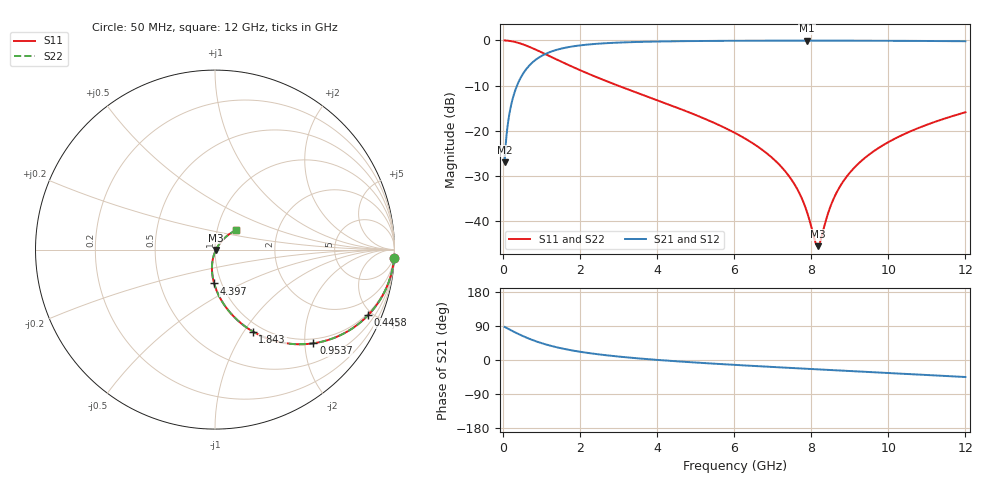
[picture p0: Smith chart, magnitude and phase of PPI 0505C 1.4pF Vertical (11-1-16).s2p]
# GHz S MA R 50
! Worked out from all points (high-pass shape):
!   1601 points, 50 MHz to 12 GHz, reference 50 ohm
!   highest |S21| = -0.05 dB at 7.892 GHz (marker M1); lowest = -27.0 dB at 50 MHz (marker M2)
!   |S21| within 3 dB of the highest: 1.096 GHz to end of sweep
!   lowest |S11| = -45.6 dB at 8.169 GHz (marker M3), VSWR 1.01, Z = 50.5 - j0.231 ohm
!   |S11| at or under -10 dB: 2.985 GHz to end of sweep
!   |S22| runs from -45.6 to 0.0 dB; largest |S21 - S12| = 0
!   S11 on the Smith chart (normalised r, x): 50 MHz: 1, -42; 445.8 MHz: 0.89, -4.72; 953.7 MHz: 0.89, -2.19; 1.843 GHz: 0.90, -1.10; 4.397 GHz: 0.92, -0.36; 12 GHz: 1.23, +0.27
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0.05  0.999 -2.7  0.04464 87.3  0.04464 87.3  0.999 -2.7
0.1470937  0.9914 -7.9  0.1304 82.0  0.1304 82.0  0.9914 -7.9
0.2068437  0.9833 -11.1  0.1818 78.9  0.1818 78.9  0.9833 -11.1
0.4458437  0.9284 -23.1  0.3708 66.8  0.3708 66.8  0.9284 -23.1
0.9537187  0.7569 -43.6  0.652 46.3  0.652 46.3  0.7569 -43.6
1.8425  0.5026 -65.2  0.862 24.5  0.862 24.5  0.5026 -65.2
2.044156  0.4605 -68.5  0.885 21.1  0.885 21.1  0.4605 -68.5
2.880656  0.329 -79.1  0.9411 10.4  0.9411 10.4  0.329 -79.1
4.038312  0.2149 -89.0  0.9728 0.0  0.9728 0.0  0.2149 -89.0
4.396813  0.1883 -91.5  0.9781 -2.6  0.9781 -2.6  0.1883 -91.5
6.025  0.09433 -100.3  0.9908 -12.9  0.9908 -12.9  0.09433 -100.3
7.234938  0.0394 -102.6  0.9939 -19.7  0.9939 -19.7  0.0394 -102.6
7.615844  0.0235 -99.4  0.9942 -21.8  0.9942 -21.8  0.0235 -99.4
7.892188  0.01256 -89.1  0.9943 -23.2  0.9943 -23.2  0.01256 -89.1
8.019156  0.008107 -74.1  0.9943 -23.9  0.9943 -23.9  0.008107 -74.1
8.168531  0.00525 -25.8  0.9942 -24.7  0.9942 -24.7  0.00525 -25.8
8.243219  0.006049 4.1  0.9942 -25.1  0.9942 -25.1  0.006049 4.1
8.541969  0.01605 43.7  0.9939 -26.6  0.9939 -26.6  0.01605 43.7
8.848187  0.02806 50.4  0.9935 -28.2  0.9935 -28.2  0.02806 50.4
9.341125  0.04781 52.3  0.9925 -30.8  0.9925 -30.8  0.04781 52.3
10.01331  0.07511 51.0  0.9905 -34.3  0.9905 -34.3  0.07511 51.0
12  0.1599 42.6  0.9793 -44.9  0.9793 -44.9  0.1599 42.6
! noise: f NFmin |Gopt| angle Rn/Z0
0.05  0.0009862  0.9602  1.65  0.005588
1.372  0.005843  0.7679  5.843  0.005111
2.701  0.009228  0.7174  9.506  0.006414
4.031  0.01222  0.6875  13.25  0.007501
5.36  0.01504  0.6675  16.98  0.008501
6.682  0.01777  0.6539  20.64  0.009475
8.012  0.02051  0.6449  24.27  0.01048
9.341  0.0233  0.6396  27.82  0.01153
10.67  0.02619  0.6375  31.3  0.01268
12  0.02922  0.6383  34.71  0.01395
